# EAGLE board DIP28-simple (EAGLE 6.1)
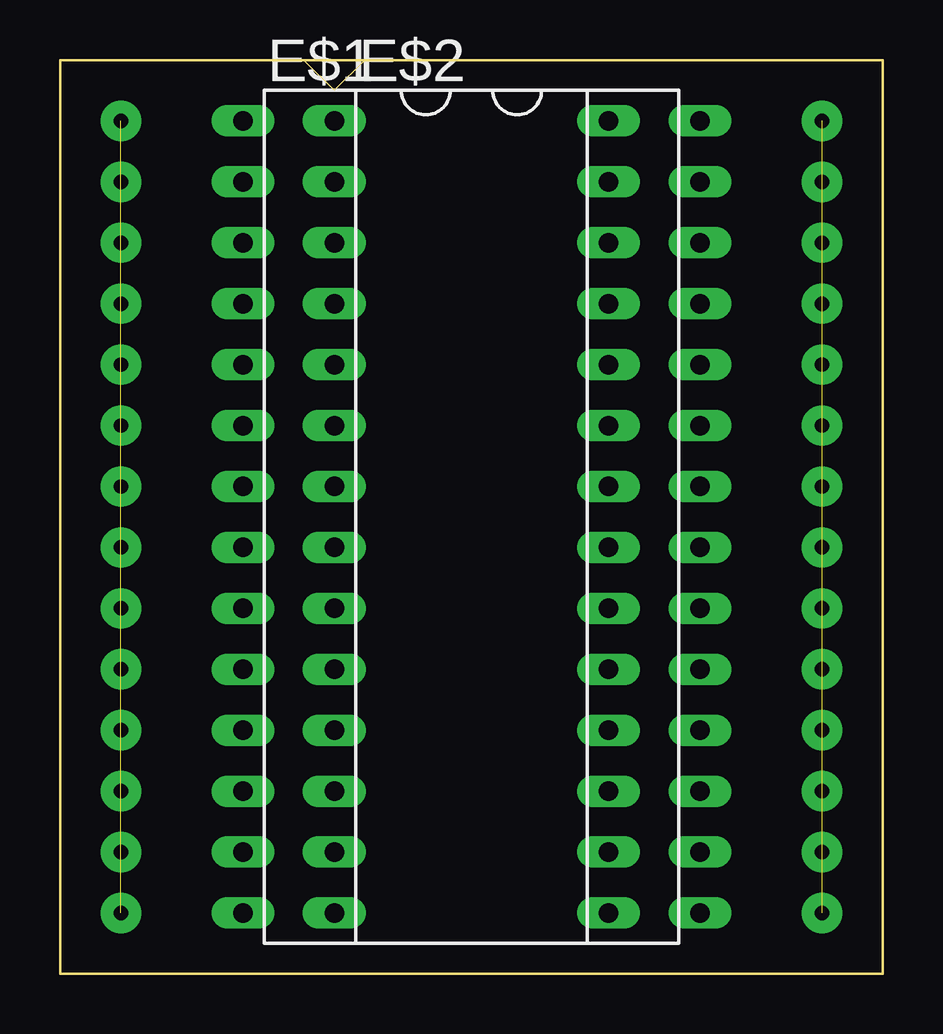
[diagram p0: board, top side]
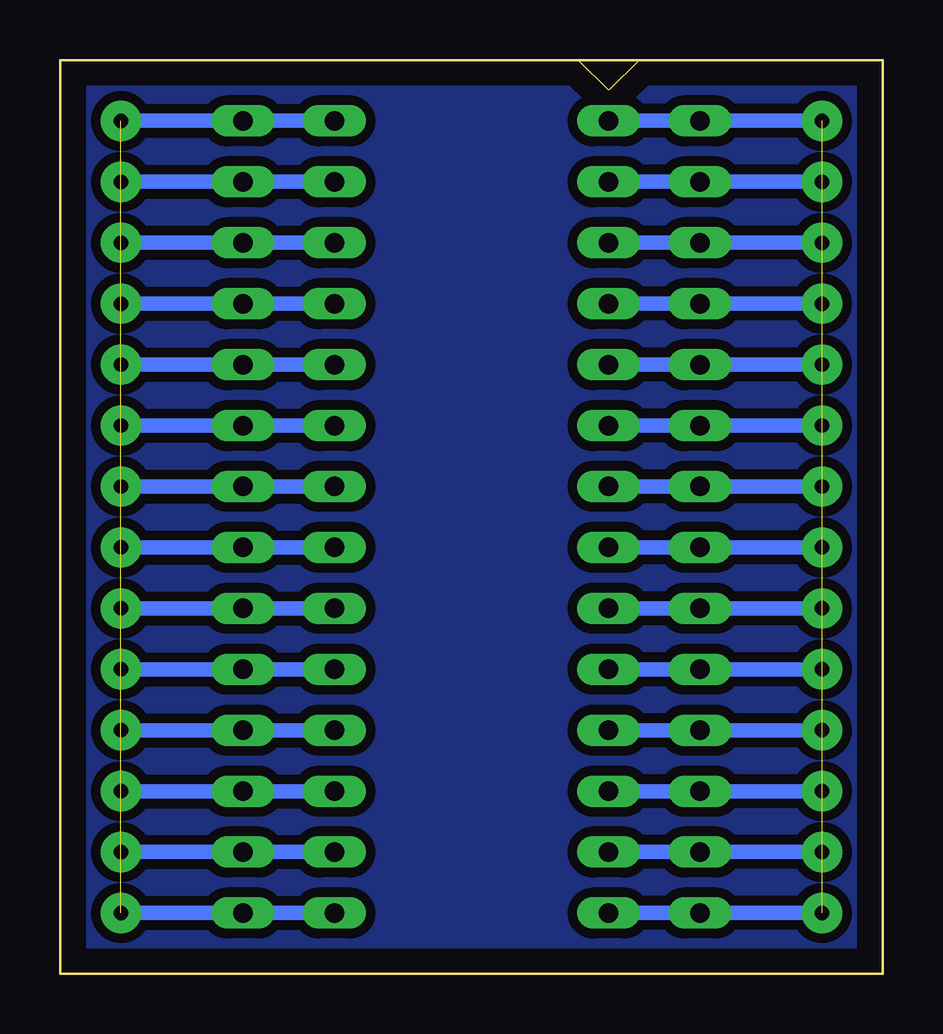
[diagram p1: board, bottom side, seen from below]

Size 34.29 x 38.1 mm. Coordinates in mm from the lower left corner, seen from the top.
Outline: 0,38.1 34.29,38.1 34.29,0 0,0 0,38.1
Copper layers (1*16): Top 0.035mm / dielectric 1.5mm / Bottom 0.035mm
Design rules: minimum track width 10mil, minimum drill 24mil, track to track 8mil, track to pad 8mil, pad to pad 8mil, via to via 8mil, smd to smd 8mil, copper to edge 40mil, drill to drill 8mil, minimum pad ring 10mil, minimum via ring 8mil, stop-mask expansion 4mil, vias tented up to drill 0mil, thermal gap 10mil

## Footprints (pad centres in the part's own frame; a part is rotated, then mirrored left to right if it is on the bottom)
DIL28 = drill 0.813 long: 1 -16.51,-7.62; 2 -13.97,-7.62; 3 -11.43,-7.62; 4 -8.89,-7.62; 5 -6.35,-7.62; 6 -3.81,-7.62; 7 -1.27,-7.62; 8 1.27,-7.62; 9 3.81,-7.62; 10 6.35,-7.62; 11 8.89,-7.62; 12 11.43,-7.62; 13 13.97,-7.62; 14 16.51,-7.62; 15 16.51,7.62; 16 13.97,7.62; 17 11.43,7.62; 18 8.89,7.62; 19 6.35,7.62; 20 3.81,7.62; 21 1.27,7.62; 22 -1.27,7.62; 23 -3.81,7.62; 24 -6.35,7.62; 25 -8.89,7.62; 26 -11.43,7.62; 27 -13.97,7.62; 28 -16.51,7.62

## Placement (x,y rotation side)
E$1  [DIL28]  15.24,19.05 270 top
E$2  [DIL28]  19.05,19.05 270 top

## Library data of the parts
E$1 E$2 = ic-package

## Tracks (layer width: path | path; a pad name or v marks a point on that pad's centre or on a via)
S$1  (via drill 0.6 pad 1.68)  (13 unrouted)
  Bottom 0.61: v2.54,35.56 11.43,35.56 | 2.54,33.02 11.43,33.02 | 2.54,30.48 11.43,30.48 | 2.54,27.94 11.43,27.94 | 2.54,25.4 11.43,25.4 | 2.54,22.86 11.43,22.86 | 2.54,20.32 11.43,20.32 | 2.54,17.78 11.43,17.78 | 2.54,15.24 11.43,15.24 | 2.54,12.7 11.43,12.7 | 2.54,10.16 11.43,10.16 | 2.54,7.62 11.43,7.62 | 2.54,5.08 11.43,5.08 | 2.54,2.54 11.43,2.54
S$2  (via drill 0.6 pad 1.68)
  other vias: 2.54,33.02
S$3  (via drill 0.6 pad 1.68)
  other vias: 2.54,30.48
S$4  (via drill 0.6 pad 1.68)
  other vias: 2.54,27.94
S$5  (via drill 0.6 pad 1.68)
  other vias: 2.54,25.4
S$6  (via drill 0.6 pad 1.68)
  other vias: 2.54,22.86
S$7  (via drill 0.6 pad 1.68)
  other vias: 2.54,20.32
S$8  (via drill 0.6 pad 1.68)
  other vias: 2.54,17.78
S$9  (via drill 0.6 pad 1.68)
  other vias: 2.54,15.24
S$10  (via drill 0.6 pad 1.68)
  other vias: 2.54,12.7
S$11  (via drill 0.6 pad 1.68)
  other vias: 2.54,10.16
S$12  (via drill 0.6 pad 1.68)
  other vias: 2.54,7.62
S$13  (via drill 0.6 pad 1.68)
  other vias: 2.54,5.08
S$14  (via drill 0.6 pad 1.68)
  other vias: 2.54,2.54
S$21  (13 unrouted)
  Bottom 0.61: 31.75,2.54 22.86,2.54 | 31.75,5.08 22.86,5.08 | 31.75,7.62 22.86,7.62 | 31.75,10.16 22.86,10.16 | 31.75,12.7 22.86,12.7 | 31.75,15.24 22.86,15.24 | 31.75,17.78 22.86,17.78 | 31.75,20.32 22.86,20.32 | 31.75,22.86 22.86,22.86 | 31.75,25.4 22.86,25.4 | 31.75,27.94 22.86,27.94 | 31.75,30.48 22.86,30.48 | 31.75,33.02 22.86,33.02 | 31.75,35.56 22.86,35.56
S$27  (via drill 0.6 pad 1.68)
  other vias: 31.75,2.54
S$28  (via drill 0.6 pad 1.68)
  other vias: 31.75,5.08
S$29  (via drill 0.6 pad 1.68)
  other vias: 31.75,7.62
S$30  (via drill 0.6 pad 1.68)
  other vias: 31.75,10.16
S$31  (via drill 0.6 pad 1.68)
  other vias: 31.75,12.7
S$32  (via drill 0.6 pad 1.68)
  other vias: 31.75,15.24
S$33  (via drill 0.6 pad 1.68)
  other vias: 31.75,17.78
S$34  (via drill 0.6 pad 1.68)
  other vias: 31.75,20.32
S$35  (via drill 0.6 pad 1.68)
  other vias: 31.75,22.86
S$36  (via drill 0.6 pad 1.68)
  other vias: 31.75,25.4
S$37  (via drill 0.6 pad 1.68)
  other vias: 31.75,27.94
S$38  (via drill 0.6 pad 1.68)
  other vias: 31.75,30.48
S$39  (via drill 0.6 pad 1.68)
  other vias: 31.75,33.02
S$40  (via drill 0.6 pad 1.68)
  other vias: 31.75,35.56
S$41
  pour Bottom (isolate 0.406): 0,38.1 34.29,38.1 34.29,0 0,0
